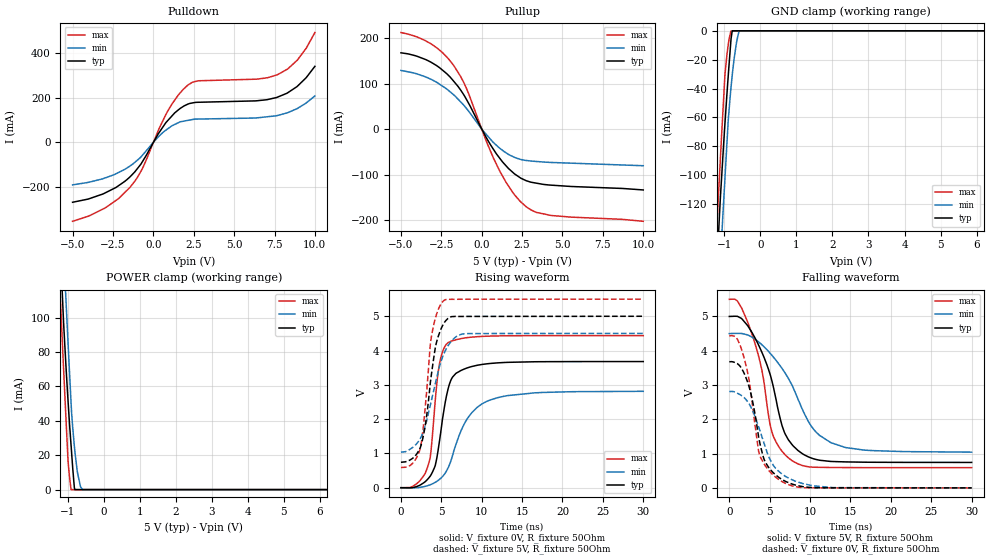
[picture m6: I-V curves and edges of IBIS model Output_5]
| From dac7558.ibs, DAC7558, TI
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|   TRISTATE OUTPUT 5.0V Model
[Model]   Output_5
Model_type   3-state
Polarity   Non-Inverting
Enable   Active-High
Vmeas = 2.5
Vref = 2.5
Cref = 15pF
Rref = 50
|   typ   min   max
|   (nom PVT)   (fast PVT)  (slow PVT)
|Average
C_comp   9.698e-12   9.323e-12   1.032e-11
|ON state : BUFFER OUTPUT TURNED HIGH
|C_comp   1.835e-11   1.762e-11   1.958e-11
|OFF state: BUFFER in HIGH IMPEDANCE for IOs and 3-state,
|This is BUFFER in LOW state for OUTPUT only type
|C_comp   1.041e-12   1.030e-12   1.062e-12
|Where  nom PVT is Nominal Process, 5.0V, 25C
|   fast PVT is Strong Process, 5.5V, -40C
|   slow PVT is Weak Process, 4.5V, 105C
[Voltage Range]   5   4.5   5.5
|Ambient Temperature   25   105   -40
|Junction Temperature
[Temperature Range]   25   105   -40
[Pullup Reference]   5   4.5   5.5
[Pulldown Reference]   0   0   0
[Power Clamp Reference]   5   4.5   5.5
[GND Clamp Reference]   0   0   0
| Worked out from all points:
|   slope of the pulldown table from 0 to 0.75 V, typ, clamps not added: 8.76 ohm
|   slope of the pullup table from 0 to 0.75 V, typ, clamps not added: 16.4 ohm
|   GND clamp passes 1 mA (typ) near -0.79 V on its own axis
|   POWER clamp passes 1 mA (typ) near -0.81 V on its own axis
|   falling waveform, V_fixture 5V, R_fixture 50Ohm: 20-80 % time 3.21ns typ, 4.87ns min, 2.59ns max; typ from 5 V to 0.742 V
|   rising waveform, V_fixture 0V, R_fixture 50Ohm: 20-80 % time 1.58ns typ, 3.24ns min, 1.09ns max; typ from 0 V to 3.68 V
|   rising waveform, V_fixture 5V, R_fixture 50Ohm: 20-80 % time 1.47ns typ, 2.23ns min, 1.18ns max; typ from 0.742 V to 5 V
|   falling waveform, V_fixture 0V, R_fixture 50Ohm: 20-80 % time 2.04ns typ, 2.88ns min, 1.79ns max; typ from 3.68 V to 0 V
[Pulldown]
|   Voltage   I(typ)   I(min)   I(max)
-5V       -267.1mA   -189.5mA   -352.1mA
-2.982V   -225.3mA   -158.4mA   -292.5mA
-1.442V   -153.4mA   -105.3mA   -200.3mA
-677mV    -85.94mA   -57.19mA   -116.5mA
918mV     99.7mA     62.15mA    143.3mA
1.528V    144mA      87.32mA    210.1mA
2.144V    171.2mA    98.48mA    256.4mA
2.788V    179.2mA    104.3mA    275.1mA
6.412V    186mA      109.7mA    282.4mA
7.672V    201.8mA    120mA      301.8mA
8.909V    250.3mA    151.4mA    367.1mA
10V       339.6mA    207.6mA    490.4mA
[GND Clamp]
|   Voltage   I(typ)   I(min)   I(max)
-5V       -2.205A    -2.192A    -2.236A
-1.26V    -188mA     -229.8mA   -160.3mA
-1.193V   -155.3mA   -197.3mA   -127.4mA
-1.115V   -117.2mA   -161.3mA   -90.16mA
-1.044V   -88.15mA   -128.8mA   -57.35mA
-979.5mV  -62.28mA   -100.1mA   -28.9mA
-896mV    -32.05mA   -63.15mA   -10.11mA
-815mV    -5.5mA     -38.87mA   -140.6uA
-783.5mV  -96.35uA   -30.94mA   0A
-671mV    0A         -9.235mA   0A
-580mV    0A         0A         0A
10V       0A         0A         0A
[Pullup]
|   Voltage   I(typ)   I(min)   I(max)
-5V       167.6mA    128.9mA    212.1mA
-3.13V    146.8mA    109.3mA    187.2mA
-2.388V   128.3mA    93.36mA    166.7mA
-1.744V   105.5mA    75.59mA    140.2mA
-963mV    66.32mA    46.06mA    90.9mA
335mV     -22mA      -13.97mA   -31.06mA
1.089V    -62.87mA   -41.34mA   -90.43mA
1.919V    -94.97mA   -60.27mA   -139.1mA
2.749V    -113.4mA   -69mA      -170.6mA
3.388V    -118.9mA   -71.24mA   -183.2mA
4.301V    -123.3mA   -73.38mA   -189.9mA
10V       -133.8mA   -80.58mA   -202.7mA
[POWER Clamp]
|   Voltage   I(typ)   I(min)   I(max)
-5V       2.172A     2.165A     2.196A
-1.238V   156.6mA    197mA      127.6mA
-1.193V   135.2mA    175.6mA    106.9mA
-1.117V   98.92mA    141.7mA    72.04mA
-1.04V    69.28mA    107.3mA    38.32mA
-985mV    50.15mA    83.67mA    15.58mA
-902.5mV  24.99mA    49.47mA    0A
-810.5mV  630.6uA    24.5mA     0A
-725mV    0A         9.587mA    0A
-644mV    0A         1.801mA    0A
-585mV    0A         0A         0A
10V       0A         0A         0A
[Ramp]
R_load = 50
|   typ   min   max
dV/dt_r   2.2075/1.57345e-09   1.68678/3.21645e-09   2.66162/1.0945e-09
dV/dt_f   2.55483/3.21217e-09   2.0749/4.87249e-09   2.94625/2.5909e-09
[Falling Waveform]
V_fixture = 5V
V_fixture_min = 4.5V
V_fixture_max = 5.5V
R_fixture = 50Ohm
C_fixture = 0F
|   Time   V(typ)   V(min)   V(max)
0s        5V         4.5V       5.5V
1.475ns   4.946V     4.504V     5.267V
3.475ns   4.238V     4.288V     3.973V
4.175ns   3.877V     4.144V     3.254V
5.35ns    3.048V     3.846V     1.573V
6.525ns   1.818V     3.485V     1.07V
7.725ns   1.274V     3.014V     801.3mV
10.15ns   870.7mV    1.801V     606.6mV
12.67ns   769.7mV    1.31V      594.5mV
30ns      741.9mV    1.042V     589.6mV
[Rising Waveform]
V_fixture = 0V
V_fixture_min = 0V
V_fixture_max = 0V
R_fixture = 50Ohm
C_fixture = 0F
|   Time   V(typ)   V(min)   V(max)
0s        866.8pV    1.142nV    719.5pV
1.925ns   31.86mV    -691.9uV   111.9mV
3.325ns   251.3mV    60.9mV     622.8mV
3.7ns     365.7mV    93.26mV    1.031V
4.25ns    648.2mV    157.2mV    2.549V
4.725ns   1.286V     233.1mV    3.552V
5.85ns    2.894V     584.1mV    4.233V
8.125ns   3.488V     1.98V      4.375V
10.98ns   3.622V     2.552V     4.421V
30ns      3.679V     2.811V     4.436V
[Rising Waveform]
V_fixture = 5V
V_fixture_min = 4.5V
V_fixture_max = 5.5V
R_fixture = 50Ohm
C_fixture = 0F
|   Time   V(typ)   V(min)   V(max)
0s        741.9mV    1.039V     589.6mV
1.4ns     848.7mV    1.165V     699.9mV
2.4ns     1.173V     1.435V     1.143V
3.05ns    1.874V     1.838V     2.455V
3.8ns     3.35V      2.571V     4.446V
4.375ns   4.212V     3.156V     5.033V
5.35ns    4.808V     3.923V     5.465V
6.525ns   4.993V     4.344V     5.495V
8.15ns    4.996V     4.496V     5.497V
30ns      5V         4.5V       5.5V
[Falling Waveform]
|Gnd
V_fixture = 0V
V_fixture_min = 0V
V_fixture_max = 0V
R_fixture = 50Ohm
C_fixture = 0F
|   Time   V(typ)   V(min)   V(max)
0s        3.679V     2.812V     4.436V
975ps     3.627V     2.763V     4.344V
1.925ns   3.294V     2.613V     3.707V
2.75ns    2.665V     2.32V      2.647V
3.775ns   1.311V     1.68V      945mV
4.475ns   741.9mV    1.179V     636.6mV
5.3ns     475.7mV    714.4mV    402.4mV
6.325ns   274.1mV    439.9mV    211.1mV
12.85ns   523.6uV    7.285mV    198.6uV
30ns      963.7nV    14.43uV    80.38nV
